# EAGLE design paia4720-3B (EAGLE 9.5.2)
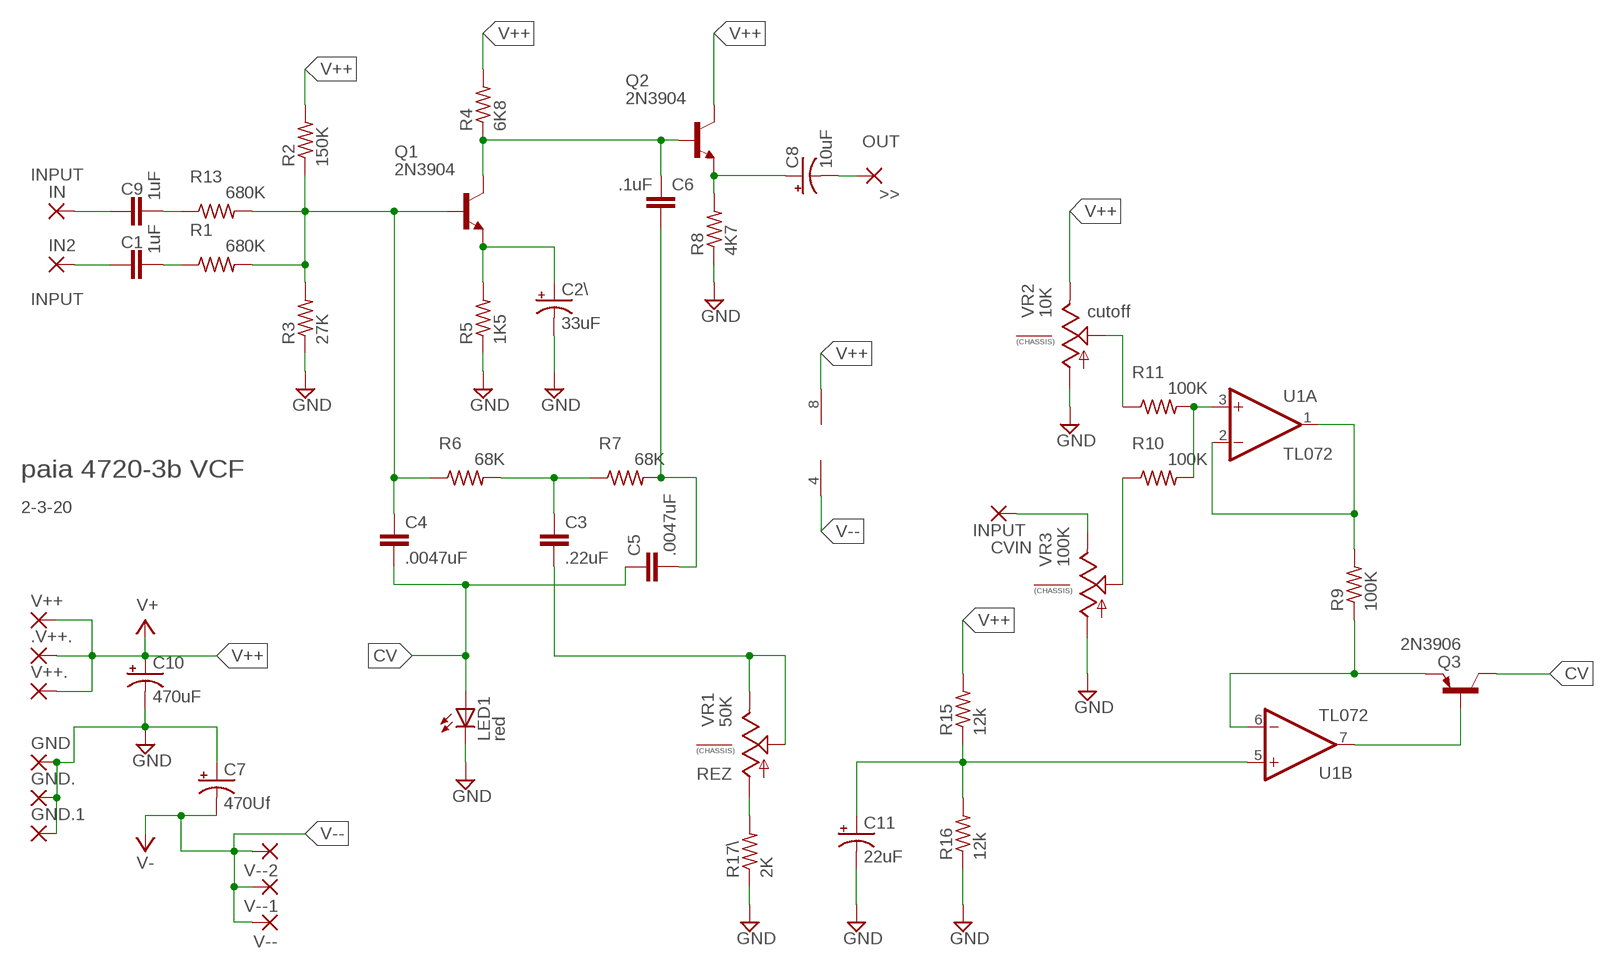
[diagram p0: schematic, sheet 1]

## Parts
.V++.  3,17/1,3  [3,17/1,3]
C1  1uF  C5/3.5  [C5B3.5]
C2\  33uF  CPOL-USE2.5-7  [E2,5-7]
C3  .22uF  C5/3.5  [C5B3.5]
C4  .0047uF  C5/3.5  [C5B3.5]
C5  .0047uF  C5/3.5  [C5B3.5]
C6  .1uF  C5/3.5  [C5B3.5]
C7  470Uf  CPOL-USE2.5-7  [E2,5-7]
C8  10uF  CPOL-USE2.5-7  [E2,5-7]
C9  1uF  C5/3.5  [C5B3.5]
C10  470uF  CPOL-USE2.5-7  [E2,5-7]
C11  22uF  CPOL-USE2.5-7  [E2,5-7]
CVIN  INPUT  3,17/1,3  [3,17/1,3]
GND  3,17/1,3  [3,17/1,3]
GND.  3,17/1,3  [3,17/1,3]
GND.1  3,17/1,3  [3,17/1,3]
IN  INPUT  3,17/1,3  [3,17/1,3]
IN2  INPUT  3,17/1,3  [3,17/1,3]
LED1  red  LED3MM  [LED3MM]
OUT  >>  3,17/1,3  [3,17/1,3]
Q1  2N3904  [TO92]
Q2  2N3904  [TO92]
Q3  2N3906  [TO92]
R1  680K  R-US_0204/7  [0204/7]
R2  150K  R-US_0204/7  [0204/7]
R3  27K  R-US_0204/7  [0204/7]
R4  6K8  R-US_0204/7  [0204/7]
R5  1K5  R-US_0204/7  [0204/7]
R6  68K  R-US_0204/7  [0204/7]
R7  68K  R-US_0204/7  [0204/7]
R8  4K7  R-US_0204/7  [0204/7]
R9  100K  R-US_0204/7  [0204/7]
R10  100K  R-US_0204/7  [0204/7]
R11  100K  R-US_0204/7  [0204/7]
R13  680K  R-US_0204/7  [0204/7]
R15  12k  R-US_0204/7  [0204/7]
R16  12k  R-US_0204/7  [0204/7]
R17\  2K  R-US_0204/7  [0204/7]
U1  TL072  [DIL08-SML]
V++  3,17/1,3  [3,17/1,3]
V++.  3,17/1,3  [3,17/1,3]
V--  3,17/1,3  [3,17/1,3]
V--1  3,17/1,3  [3,17/1,3]
V--2  3,17/1,3  [3,17/1,3]
VR1  50K  9MM_SNAP-IN_POT_CHASSIS  [9MM_SNAP-IN_POT]
VR2  10K  9MM_SNAP-IN_POT_CHASSIS  [9MM_SNAP-IN_POT]
VR3  100K  9MM_SNAP-IN_POT_CHASSIS  [9MM_SNAP-IN_POT]

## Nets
CV: C4.2 C5.1 LED1.A Q3.1(C)
GND: C2\.- C7.+ C10.- C11.- GND.1(P) GND.1.1(P) GND..1(P) LED1.K(C) R3.1 R5.1 R8.1 R16.1 R17\.1 VR2.1(A) VR3.1(A)
N$1: C9.1 IN.1(P)
N$2: R10.1 VR3.2(S)
N$3: C9.2 R13.1
N$4: C4.1 Q1.2(B) R1.2 R2.1 R3.2 R6.1 R13.2
N$5: R10.2 R11.2 U1.3(A:+IN)
N$6: C1.1 IN2.1(P)
N$7: R11.1 VR2.2(S)
N$8: C1.2 R1.1
N$9: C6.1 Q1.1(C) Q2.2(B) R4.1
N$10: C3.2 VR1.2(S) VR1.3(E)
N$11: C2\.+ Q1.3(E) R5.2
N$12: C8.+ Q2.3(E) R8.2
N$13: C8.- OUT.1(P)
N$14: C3.1 R6.2 R7.1
N$15: C5.2 C6.2 R7.2
N$16: R9.2 U1.1(A:OUT) U1.2(A:-IN)
N$20: CVIN.1(P) VR3.3(E)
N$21: R17\.2 VR1.1(A)
N$22: Q3.3(E) R9.1 U1.6(B:-IN)
N$23: Q3.2(B) U1.7(B:OUT)
N$24: C11.+ R15.1 R16.2 U1.5(B:+IN)
V++: .V++..1(P) C10.+ Q2.1(C) R2.2 R4.2 R15.2 U1.8(P:V+) V++.1(P) V++..1(P) VR2.3(E) ; supply symbol labelled V+
V--: C7.- U1.4(P:V-) V--1.1(P) V--2.1(P) V--.1(P) ; supply symbol labelled V-
Unconnected: VR1.CHASSIS1 VR1.CHASSIS2 VR2.CHASSIS1 VR2.CHASSIS2 VR3.CHASSIS1 VR3.CHASSIS2

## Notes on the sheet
- cutoff
- paia 4720-3b VCF
- 2-3-20
- REZ

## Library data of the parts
.V++. CVIN GND GND. GND.1 IN IN2 OUT V++ V++. V-- V--1 V--2 = wirepad:3,17/1,3: THROUGH-HOLE PAD
C1 C3-C6 C9 = capacitor-wima:C: CAPACITOR
C2\ C7 C8 C10 C11 = rcl:CPOL-US: POLARIZED CAPACITOR, American symbol; SPICEPREFIX: C
LED1 = adafruit:LED: LED
Q1 Q2 = transistor:2N3904: NPN TRANSISTOR
Q3 = transistor-pnp:2N3906: PNP Transistor
R1-R11 R13 R15 R16 R17\ = rcl:R-US_: RESISTOR, American symbol
U1 = MusicThingModular:TL072: Generic Dual Op Amp
VR1-VR3 = MusicThingModular:9MM_SNAP-IN_POT_CHASSIS: 9mm vertical snap-in pot, Alpha / Panasonic style, with a connection to the metal chassis for grounding

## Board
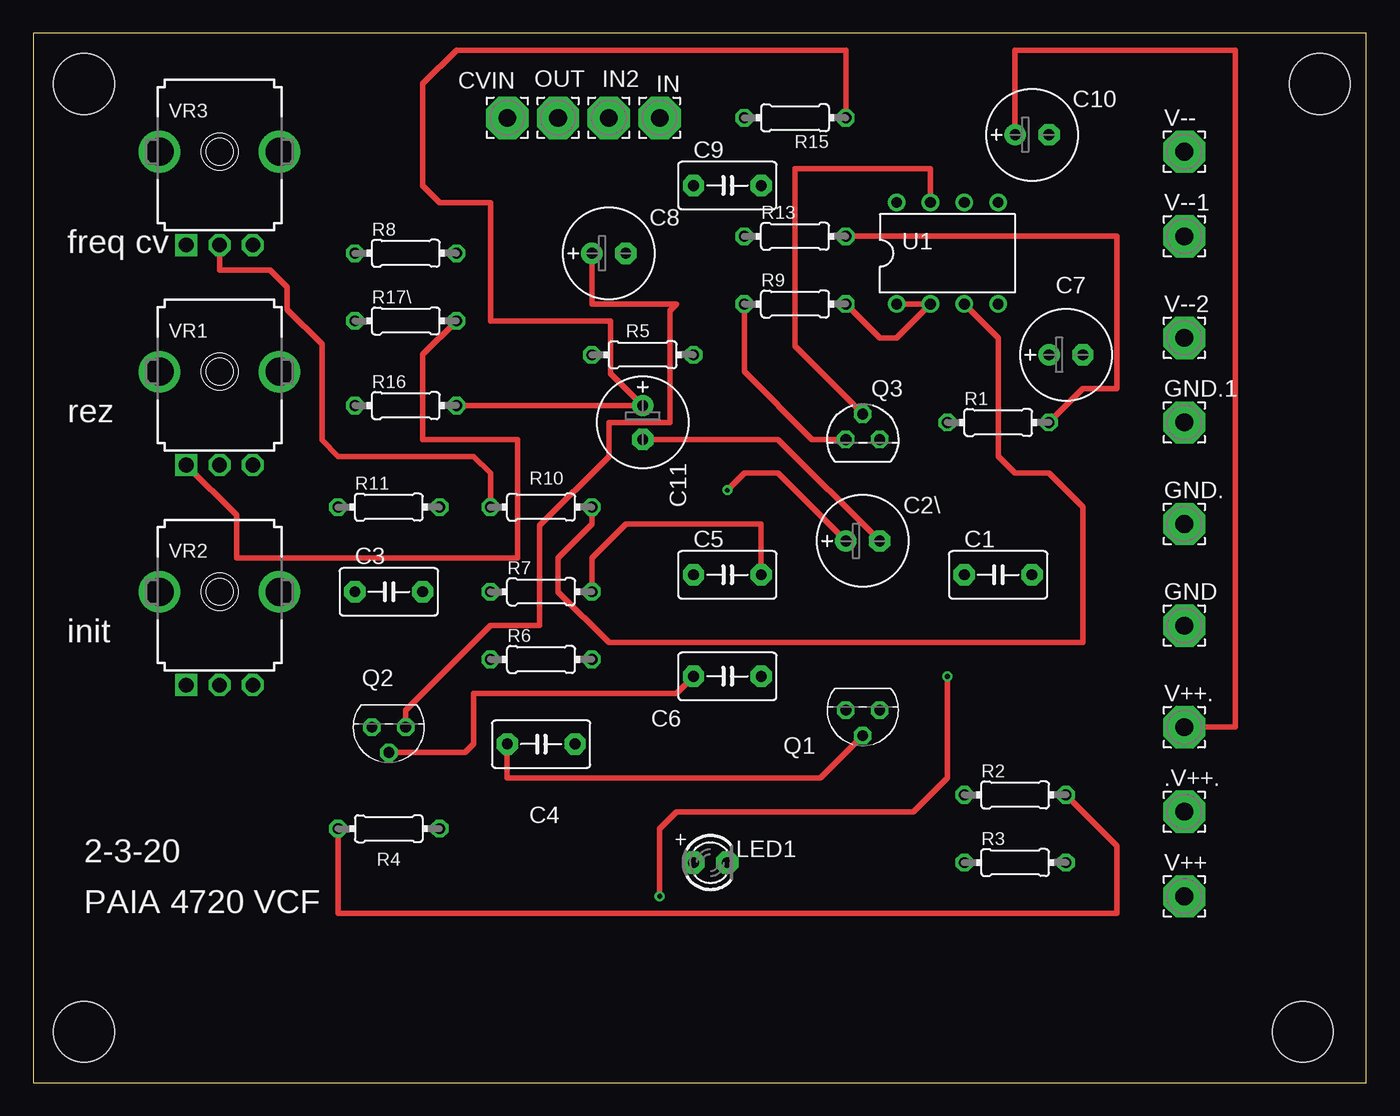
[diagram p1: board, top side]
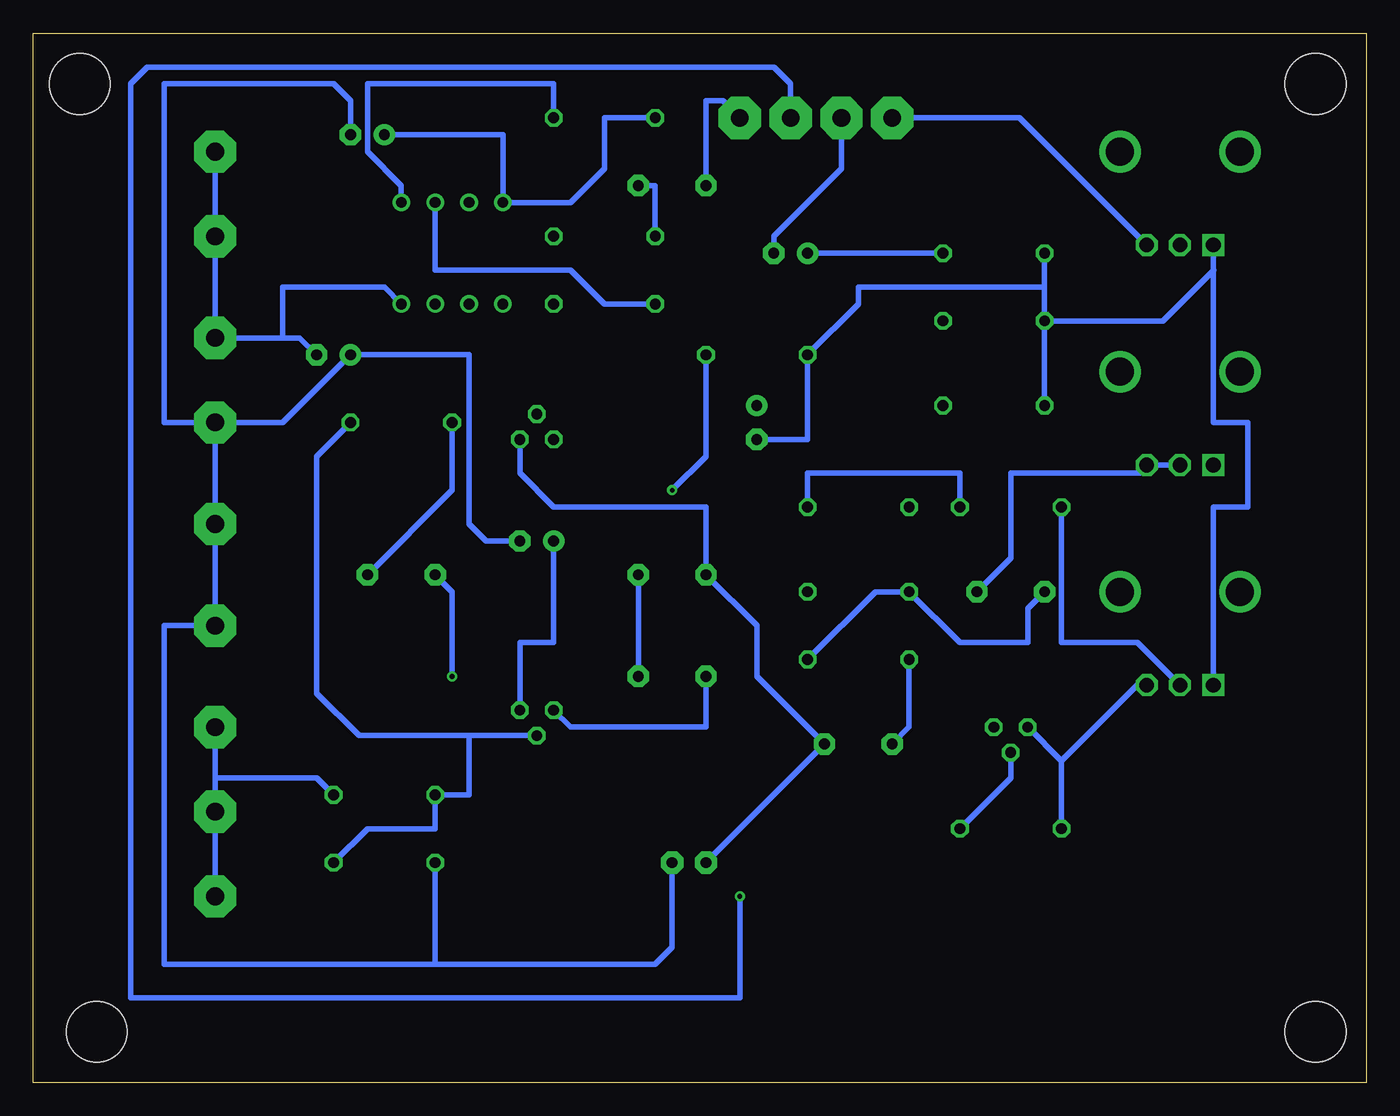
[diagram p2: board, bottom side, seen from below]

Size 100 x 78.73 mm. Coordinates in mm from the lower left corner, seen from the top.
Outline: 0,0 100,0 100,78.73 0,78.73 0,0
Copper layers (1*16): Top 0.035mm / dielectric 1.5mm / Bottom 0.035mm
Design rules "default": minimum track width 6mil, minimum drill 0.35mm, track to track 6mil, track to pad 6mil, pad to pad 6mil, via to via 6mil, smd to smd 6mil, copper to edge 40mil, drill to drill 6mil, minimum pad ring 10mil, minimum via ring 8mil, stop-mask expansion 4mil, vias tented up to drill 0mil, thermal gap 10mil
Holes 4.57 mm at 3.81,74.93 3.81,3.81 95.25,3.81 96.52,74.93

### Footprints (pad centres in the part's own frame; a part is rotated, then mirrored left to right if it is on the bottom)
3,17/1,3 = drill 1.321 pad 3.175 octagon: 1 0,0
C5B3.5 = drill 0.813 pad 1.6 octagon: 1 -2.54,0; 2 2.54,0
E2,5-7 = drill 0.813 pad 1.6: + -1.27,0 | drill 0.813 pad 1.6 octagon: - 1.27,0
LED3MM = drill 0.813 pad 1.676 octagon: A -1.27,0; K 1.27,0
TO92 = drill 0.813 octagon: 1 1.27,0; 2 0,1.905; 3 -1.27,0
0204/7 = drill 0.813 octagon: 1 -3.81,0; 2 3.81,0
DIL08-SML = drill 0.813 pad 1.27: 1 -3.81,-3.81; 2 -1.27,-3.81; 3 1.27,-3.81; 4 3.81,-3.81; 5 3.81,3.81; 6 1.27,3.81; 7 -1.27,3.81; 8 -3.81,3.81
9MM_SNAP-IN_POT = drill 1.1 square: 1 -2.5,-7 | drill 1.1 octagon: 2 0,-7; 3 2.5,-7 | drill 2.1 pad 2.794: CHASSIS1 -4.5,0; CHASSIS2 4.5,0

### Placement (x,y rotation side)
.V++.  86.36,20.32 0 top
C1  72.39,38.1 0 top
C2\  62.23,40.64 0 top
C3  26.67,36.83 0 top
C4  38.1,25.4 0 top
C5  52.07,38.1 0 top
C6  52.07,30.48 0 top
C7  77.47,54.61 0 top
C8  43.18,62.23 0 top
C9  52.07,67.31 0 top
C10  74.93,71.12 0 top
C11  45.72,49.53 270 top
CVIN  35.56,72.39 0 top
GND  86.36,34.29 0 top
GND.  86.36,41.91 0 top
GND.1  86.36,49.53 0 top
IN  46.99,72.39 0 top
IN2  43.18,72.39 0 top
LED1  50.8,16.51 0 top
OUT  39.37,72.39 0 top
Q1  62.23,27.94 180 top
Q2  26.67,26.67 180 top
Q3  62.23,48.26 0 top
R1  72.39,49.53 0 top
R2  73.66,21.59 0 top
R3  73.66,16.51 0 top
R4  26.67,19.05 180 top
R5  45.72,54.61 0 top
R6  38.1,31.75 0 top
R7  38.1,36.83 0 top
R8  27.94,62.23 0 top
R9  57.15,58.42 0 top
R10  38.1,43.18 0 top
R11  26.67,43.18 0 top
R13  57.15,63.5 0 top
R15  57.15,72.39 180 top
R16  27.94,50.8 0 top
R17\  27.94,57.15 0 top
U1  68.58,62.23 0 top
V++  86.36,13.97 0 top
V++.  86.36,26.67 0 top
V--  86.36,69.85 0 top
V--1  86.36,63.5 0 top
V--2  86.36,55.88 0 top
VR1  13.97,53.34 0 top
VR2  13.97,36.83 0 top
VR3  13.97,69.85 0 top

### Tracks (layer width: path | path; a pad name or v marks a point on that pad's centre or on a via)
CV
  Bottom 0.406: LED1.A C4.2 45.72,30.48 45.72,34.29 C5.1 49.53,43.18 60.96,43.18 63.5,45.72 Q3.1
GND
  Top 0.406: C2\.- 55.88,48.26 C11.-
  Bottom 0.406: GND.1.1 GND..1 GND.1 90.17,34.29 90.17,8.89 69.85,8.89 | 69.85,8.89 R3.1 | 69.85,8.89 53.34,8.89 52.07,10.16 LED1.K | GND.1.1 81.28,49.53 C7.+ 67.31,54.61 67.31,41.91 66.04,40.64 C2\.- | GND.1.1 90.17,49.53 90.17,74.93 77.47,74.93 76.2,73.66 C10.- | C11.- 41.91,48.26 R5.1 38.1,58.42 38.1,59.69 24.13,59.69 | R16.1 R17\.1 | R17\.1 24.13,59.69 | 24.13,59.69 R8.1 | VR3.1 11.47,61 | 11.47,61 11.43,60.96 15.24,57.15 R17\.1 | VR2.1 11.47,43.14 11.43,43.18 8.89,43.18 8.89,49.53 11.43,49.53 11.47,49.57 11.47,61
N$1
  Bottom 0.406: C9.1 49.53,73.66 48.26,73.66 IN.1
N$2
  Top 0.406: R10.1 34.29,45.72 33.02,46.99 22.86,46.99 21.65,48.2 21.65,55.4 19.05,58.01 19.05,59.69 17.78,60.96 13.97,60.96 VR3.2
N$3
  Bottom 0.406: R13.1 53.34,67.31 C9.2
N$4
  Top 0.406: Q1.2 59.05,22.86 35.56,22.86 C4.1 | R1.2 78.74,52.07 81.28,52.07 81.28,63.5 R13.2
  Bottom 0.406: Q1.2 67.31,26.04 | 67.31,26.04 75.56,26.04 78.74,29.21 78.74,46.99 R1.2 | C4.1 34.29,26.67 R6.1 | R3.2 74.93,19.05 69.85,19.05 R2.1 67.31,21.59 67.31,26.04
N$5
  Top 0.406: R10.2 41.91,41.91 39.37,39.37 39.37,36.83 43.18,33.02 78.74,33.02 78.74,43.18 76.2,45.72 73.66,45.72 72.39,46.99 72.39,55.88 U1.3
  Bottom 0.406: R10.2 41.91,45.72 30.48,45.72 R11.2
N$6  (via drill 0.35)
  Top 0.406: v46.99,13.97 46.99,19.05 48.26,20.32 66.04,20.32 68.58,22.86 v68.58,30.48
  Bottom 0.406: IN2.1 43.18,74.93 44.45,76.2 91.44,76.2 92.71,74.93 92.71,6.35 46.99,6.35 v46.99,13.97 | v68.58,30.48 68.58,36.83 C1.1
N$7
  Bottom 0.406: VR2.2 17.16,33.02 22.86,33.02 R11.1
N$8
  Bottom 0.406: C1.2 68.58,44.45 R1.1
N$9
  Top 0.406: C6.1 48.26,29.21 33.02,29.21 33.02,25.4 32.39,24.77 Q2.2
  Bottom 0.406: Q1.1 59.69,26.67 49.53,26.67 C6.1 | R4.1 26.67,22.86 Q2.2
N$10
  Bottom 0.406: C3.2 26.67,39.37 26.67,45.72 16.51,45.72 16.47,45.76 VR1.3 VR1.2
N$11  (via drill 0.35)
  Top 0.406: C2\.+ 55.88,45.72 53.34,45.72 v52.07,44.45
  Bottom 0.406: Q1.3 63.5,33.02 60.96,33.02 C2\.+ | v52.07,44.45 49.53,46.99 R5.2
N$12
  Top 0.406: Q2.3 27.94,27.94 34.29,34.29 37.97,34.29 37.97,41.78 43.18,46.99 43.18,49.53 47.75,49.53 47.75,57.91 48.26,58.42 41.91,58.42 C8.+
  Bottom 0.406: R8.2 C8.+
N$13
  Bottom 0.406: C8.- 44.45,63.5 39.37,68.58 OUT.1
N$14
  Bottom 0.406: C3.1 25.4,35.56 25.4,33.02 30.48,33.02 R7.1 36.83,36.83 R6.2
N$15
  Top 0.406: C5.2 54.61,41.91 44.45,41.91 41.91,39.37 R7.2
  Bottom 0.406: C6.2 C5.2
N$16
  Top 0.406: R9.2 63.5,55.88 64.77,55.88 U1.2 U1.1
N$20
  Bottom 0.406: VR3.3 26.01,72.39 CVIN.1
N$21
  Top 0.406: VR1.1 15.24,42.57 15.24,39.37 36.32,39.37 36.32,48.26 29.21,48.26 29.21,54.61 R17\.2
N$22
  Top 0.406: Q3.3 58.42,48.26 53.34,53.34 R9.1
  Bottom 0.406: R9.1 57.15,58.42 59.69,60.96 69.85,60.96 U1.6
N$23
  Top 0.406: U1.7 67.31,68.58 57.15,68.58 57.15,55.24 Q3.2
N$24
  Top 0.406: R16.2 C11.+ 43.31,53.21 43.31,57.15 34.29,57.15 34.29,66.04 30.48,66.04 29.21,67.31 29.21,74.93 31.75,77.47 60.96,77.47 R15.1
  Bottom 0.406: U1.5 72.39,67.31 74.93,69.85 74.93,74.93 60.96,74.93 R15.1
V++
  Top 0.406: C10.+ 73.66,77.47 90.17,77.47 90.17,26.67 V++..1 | R2.2 81.28,17.78 81.28,12.7 22.86,12.7 R4.2
  Bottom 0.406: C10.+ 64.77,71.12 U1.8 59.69,66.04 57.15,68.58 57.15,72.39 R15.2 | V++.1 .V++..1 86.36,22.86 | 86.36,22.86 V++..1 | R4.2 22.86,24.13 | 22.86,24.13 Q2.1 | VR2.3 17.16,29.83 22.86,24.13 | R2.2 78.74,22.86 86.36,22.86
V--
  Bottom 0.406: V--.1 V--1.1 V--2.1 81.28,55.88 | C7.- 80.01,55.88 81.28,55.88 | U1.4 73.66,59.69 81.28,59.69 81.28,55.88

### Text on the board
tNames: freq cv | rez | init | 2-3-20 | PAIA 4720 VCF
